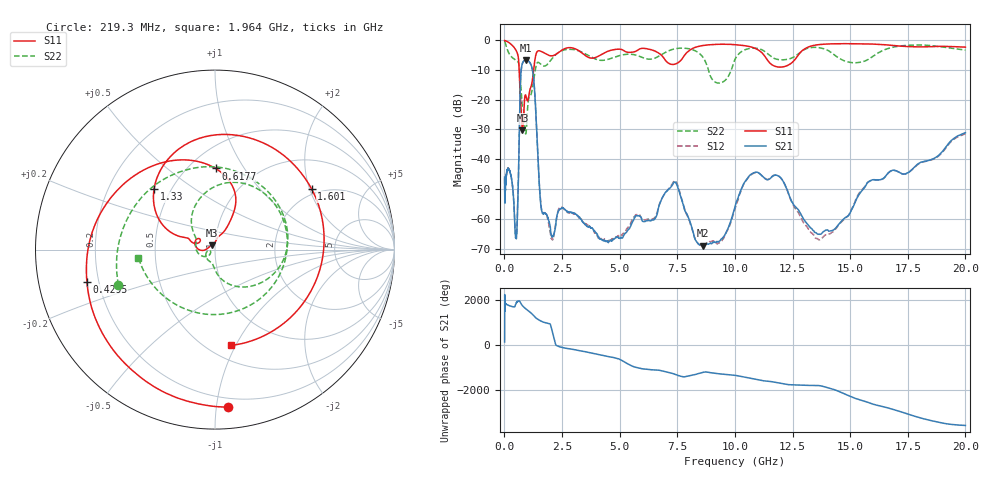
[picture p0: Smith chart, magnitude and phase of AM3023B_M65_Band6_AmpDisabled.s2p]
!Agilent Technologies,E8364B,MY43040894,A.07.50.67
!Agilent E8364B: A.07.50.67
!Date: Tuesday, October 27, 2020 10:49:40
!Correction: S11(Full 2 Port(1,2))
!S21(Full 2 Port(1,2))
!S12(Full 2 Port(1,2))
!S22(Full 2 Port(1,2))
!S2P File: Measurements: S11, S21, S12, S22:Log Frequency Sweep
# Hz S  dB  R 50
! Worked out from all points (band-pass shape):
!   3201 points, 10 MHz to 20 GHz, reference 50 ohm
!   highest |S21| = -6.85 dB at 929.5 MHz (marker M1); lowest = -68.8 dB at 8.606 GHz (marker M2)
!   |S21| within 3 dB of the highest: 733.1 MHz to 1.211 GHz (478 MHz wide, 49.2 % of centre)
!   lowest |S11| = -30.2 dB at 783.4 MHz (marker M3), VSWR 1.06, Z = 48.2 + j2.41 ohm
!   |S11| at or under -10 dB: 639.9 MHz to 1.27 GHz (630.3 MHz wide, 66 % of centre)
!   |S22| runs from -31.5 to -0.7 dB; largest |S21 - S12| = 0.0084
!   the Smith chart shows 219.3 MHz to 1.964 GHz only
!   S11 on the Smith chart (normalised r, x): 219.3 MHz: 0.14, -1.08; 429.5 MHz: 0.15, -0.12; 617.7 MHz: 0.66, +0.76; 1.33 GHz: 0.40, +0.35; 1.601 GHz: 1.82, +2.06; 1.964 GHz: 0.64, -0.96
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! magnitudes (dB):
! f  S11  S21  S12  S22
! 10 MHz  -0.3  -45.9  -46.3  -0.7
! 35.55 MHz  -0.4  -50.9  -51.4  -1.0
! 126.1 MHz  -0.7  -43.5  -43.7  -3.3
! 219.3 MHz  -1.1  -43.8  -43.6  -4.8
! 429.5 MHz  -2.7  -57.4  -57.1  -6.5
! 447.2 MHz  -2.8  -61.0  -59.6  -6.6
! 530.6 MHz  -3.9  -65.4  -64.8  -7.1
! 617.7 MHz  -6.9  -43.4  -43.6  -7.8
! 694 MHz  -19.4  -14.6  -14.7  -13.1
! 783.4 MHz  -30.2  -7.9  -7.9  -22.3
! 929.5 MHz  -18.6  -6.8  -6.9  -31.5
! 1.33 GHz  -6.4  -19.4  -19.4  -10.7
! 1.59 GHz  -3.9  -55.8  -55.6  -8.3
! 1.601 GHz  -3.9  -56.4  -56.2  -8.4
! 1.964 GHz  -5.3  -61.5  -63.5  -7.3
! 5.639 GHz  -4.1  -59.6  -59.2  -5.0
! 7.358 GHz  -8.3  -47.7  -47.2  -3.1
! 8.606 GHz  -2.0  -68.8  -69.0  -5.8
! 9.352 GHz  -1.5  -67.2  -67.8  -14.5
! 10.91 GHz  -3.0  -44.3  -44.4  -2.9
! 13.94 GHz  -1.5  -63.6  -65.2  -3.2
! 20 GHz  -2.5  -31.1  -31.4  -3.5
